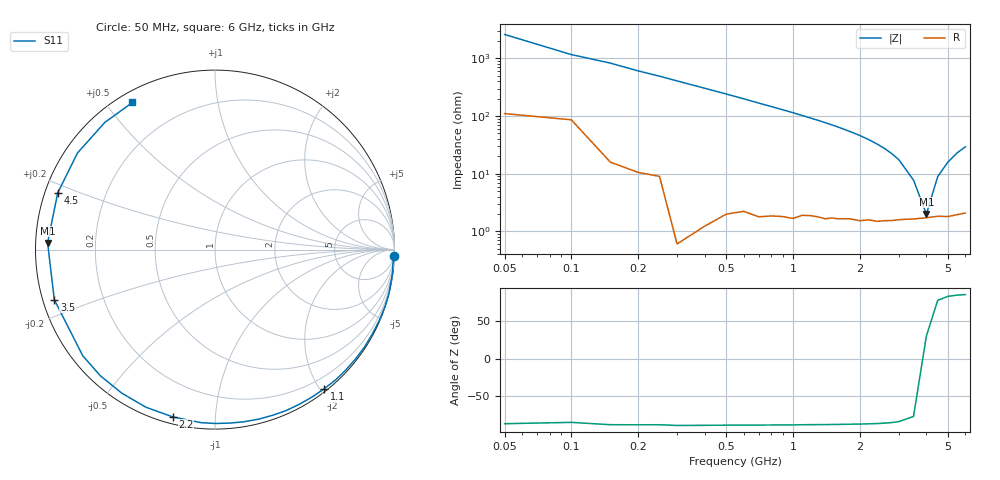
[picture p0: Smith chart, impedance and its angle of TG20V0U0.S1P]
! SIEMENS Discrete & RF Semiconductors
! BAT64
! Si Schottky Diode in SOT23
! VR = 20 V
! S-Parameters:  February  1997
# GHz  S  MA  R  50
!  f  S11
! GHz  MAG  ANG
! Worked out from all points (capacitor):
!   34 points, 50 MHz to 6 GHz, reference 50 ohm
!   read as one part to ground: C = 1.28 pF near 50 MHz
!   lowest |Z| = 2 ohm at 4 GHz (marker M1)
!   series resonance near 3.942 GHz, so ESL is about 1.3 nH
!   S11 on the Smith chart (normalised r, x): 50 MHz: 2, -52; 1.1 GHz: 0.04, -2.05; 2.2 GHz: 0.03, -0.78; 3.5 GHz: 0.03, -0.15; 4.5 GHz: 0.04, +0.17; 6 GHz: 0.04, +0.58
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0.05  0.9984 -2.2
0.1  0.9937 -4.9
0.15  0.9977 -6.9
0.3  0.9996 -14.0
0.4  0.9987 -18.7
0.5  0.9967 -23.4
0.6  0.9947 -28.2
0.7  0.9942 -33.1
0.8  0.9923 -37.8
1  0.9893 -47.2
1.1  0.9855 -52.0
1.2  0.9832 -56.7
1.4  0.9805 -66.2
1.6  0.9755 -75.6
1.7  0.9726 -80.5
1.9  0.9687 -89.9
2  0.9674 -94.6
2.2  0.9613 -104.2
2.4  0.9589 -113.7
2.6  0.9536 -123.0
2.8  0.9497 -132.3
3  0.9447 -141.3
3.5  0.9378 -162.7
4  0.9333 177.7
4.5  0.9315 160.2
5  0.9363 144.9
5.5  0.9375 130.9
6  0.9399 119.3
